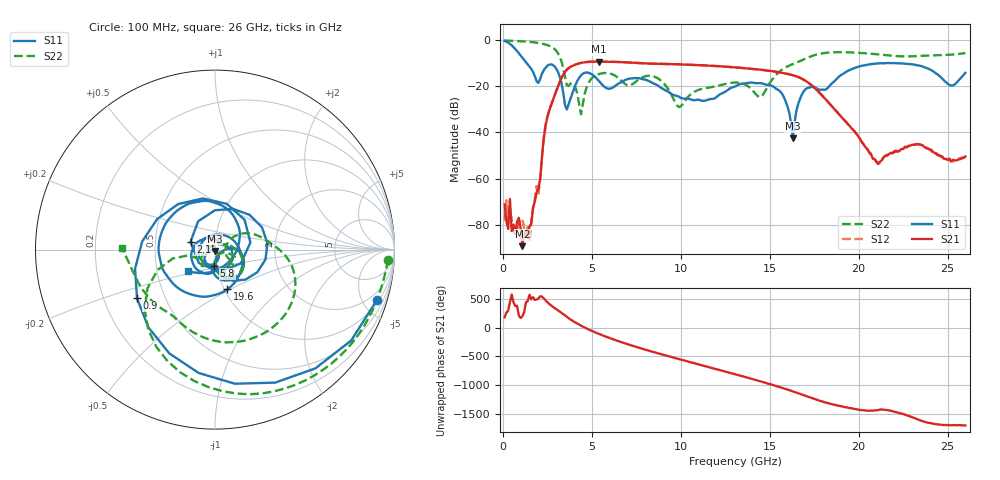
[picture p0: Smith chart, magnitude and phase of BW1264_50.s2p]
!Keysight Technologies,N5245B,MY57181159,A.13.60.06
!Date: Friday, December 18, 2020 23:54:44
!Correction: S11(Full 2 Port(1,2))
!S21(Full 2 Port(1,2))
!S12(Full 2 Port(1,2))
!S22(Full 2 Port(1,2))
!S2P File: Measurements: S11, S21, S12, S22:
# Hz S  dB  R 50
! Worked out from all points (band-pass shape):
!   260 points, 100 MHz to 26 GHz, reference 50 ohm
!   highest |S21| = -9.45 dB at 5.4 GHz (marker M1); lowest = -89.1 dB at 1.1 GHz (marker M2)
!   |S21| within 3 dB of the highest: 3.666 GHz to 13.85 GHz (10.18 GHz wide, 116 % of centre)
!   lowest |S11| = -42.5 dB at 16.3 GHz (marker M3), VSWR 1.02, Z = 49.8 - j0.708 ohm
!   |S11| at or under -10 dB: 1.328 GHz to end of sweep
!   |S22| runs from -32.2 to -0.3 dB; largest |S21 - S12| = 0.00044
!   S11 on the Smith chart (normalised r, x): 100 MHz: 1.21, -6.38; 900 MHz: 0.35, -0.25; 2.1 GHz: 0.76, +0.07; 5.8 GHz: 0.97, -0.18; 19.6 GHz: 1.03, -0.48; 26 GHz: 0.72, -0.18
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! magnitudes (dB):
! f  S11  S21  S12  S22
! 100 MHz  -0.5  -71.1  -78.1  -0.3
! 200 MHz  -0.8  -78.3  -69.4  -0.4
! 900 MHz  -5.8  -76.9  -79.1  -0.6
! 1.1 GHz  -7.8  -89.1  -77.4  -0.7
! 1.5 GHz  -11.6  -80.5  -87.2  -0.9
! 2.1 GHz  -16.9  -60.2  -60.0  -1.5
! 2.4 GHz  -12.1  -37.1  -37.2  -2.1
! 2.9 GHz  -11.4  -24.2  -24.3  -4.0
! 3.6 GHz  -30.1  -12.9  -12.9  -19.7
! 4.5 GHz  -14.7  -9.8  -9.8  -27.6
! 5.4 GHz  -17.8  -9.5  -9.5  -14.8
! 5.8 GHz  -20.8  -9.5  -9.5  -14.4
! 8.8 GHz  -20.2  -10.4  -10.4  -17.1
! 9.9 GHz  -24.6  -10.6  -10.6  -29.1
! 13.1 GHz  -20.0  -12.0  -12.0  -18.4
! 14.5 GHz  -18.8  -13.0  -12.9  -24.7
! 15.6 GHz  -22.4  -14.1  -14.1  -13.4
! 16.3 GHz  -42.5  -15.3  -15.3  -10.5
! 17.4 GHz  -20.3  -20.0  -20.0  -6.9
! 19.6 GHz  -12.7  -38.2  -38.3  -5.5
! 21.7 GHz  -10.0  -49.4  -49.1  -6.8
! 26 GHz  -14.3  -50.4  -50.8  -5.7
